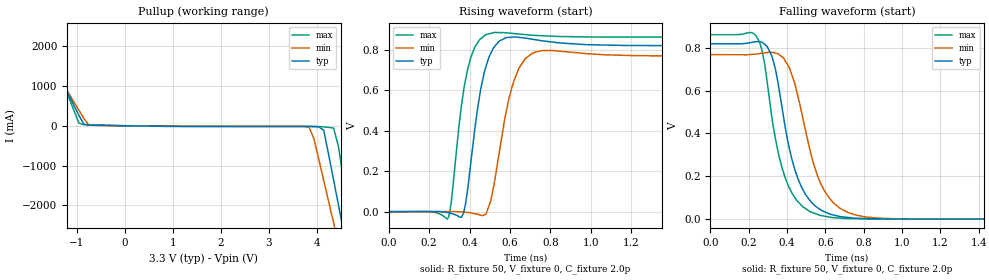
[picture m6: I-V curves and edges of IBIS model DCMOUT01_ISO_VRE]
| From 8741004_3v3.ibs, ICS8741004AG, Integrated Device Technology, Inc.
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[Model]  DCMOUT01_ISO_VRE
Model_type Open_source
Polarity  Non-Inverting
Vmeas= .323
Rref = 50
Cref = 0
Vref = 0
|Variable   typ   min   max
C_comp   2p   1.5p   2.5p
|Variable   typ   min   max
[Voltage Range]   3.3   3.135   3.465
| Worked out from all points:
|   slope of the pullup table from 0 to 0.495 V, typ, clamps not added: 57.4 ohm
|   rising waveform, R_fixture 50, V_fixture 0, C_fixture 2.0p: 20-80 % time 68.9ps typ, 85.7ps min, 65.1ps max; typ from 0 V to 0.82 V
|   falling waveform, R_fixture 50, V_fixture 0, C_fixture 2.0p: 20-80 % time 119ps typ, 137ps min, 110ps max; typ from 0.82 V to 0 V
|  Voltage   I(typ)   I(min)   I(max)
[Pullup]
-3.3V     5.929A     5.106A     7.3A
-2.075V   2.966A     2.639A     3.52A
-1.769V   2.226A     2.023A     2.576A
-952.6mV  259.6mA    387.7mA    67.22mA
-850.5mV  40.66mA    183.8mA    26.27mA
3.844V    -17.3mA    -33.95mA   -17.33mA
4.151V    -116.4mA   -1.378A    -29.1mA
4.355V    -1.355A    -2.431A    -58.99mA
4.559V    -2.622A    -3.486A    -1.33A
4.661V    -3.257A    -4.014A    -2.14A
4.763V    -3.891A    -4.542A    -2.95A
6.6V      -15.32A    -14.06A    -17.53A
|  Voltage   I(typ)   I(min)   I(max)
[Ramp]
|   typ   min   max
dV/dt_r   0.680/0.118n   0.637/0.141n   0.718/0.108n
dV/dt_f   0.680/0.198n   0.637/0.226n   0.718/0.180n
R_load =   50.0000
[Rising Waveform]
R_fixture = 50
V_fixture = 0
C_fixture = 2.0p
| Time   typ   min   max
0s        1.402nV    4.01nV     367.5pV
297.2ps   -5.136mV   575uV      -25.12mV
370.9ps   -5.979mV   -1.874mV   596.9mV
426ps     405.7mV    -9.617mV   811.8mV
480.8ps   714mV      -11.24mV   874.1mV
506.1ps   783.3mV    56.91mV    880.7mV
547.7ps   842.7mV    298mV      884.4mV
616.9ps   862.1mV    638.7mV    879.5mV
713.2ps   851mV      783.6mV    870.8mV
2ns       819.7mV    768.5mV    861.9mV
[Falling Waveform]
R_fixture = 50
V_fixture = 0
C_fixture = 2.0p
| Time   typ   min   max
0s        819.6mV    768.4mV    861.9mV
236.8ps   829mV      771mV      858.6mV
297.2ps   805.7mV    778.4mV    636mV
339.5ps   701mV      776.1mV    376.7mV
389.8ps   433.6mV    741mV      195.1mV
455.5ps   192.6mV    579.7mV    82.79mV
521.7ps   84.34mV    315.8mV    33.94mV
616.9ps   25.88mV    102.3mV    10.07mV
756ps     4.142mV    19.3mV     1.608mV
2ns       287.7pV    5.065nV    462.5pV
